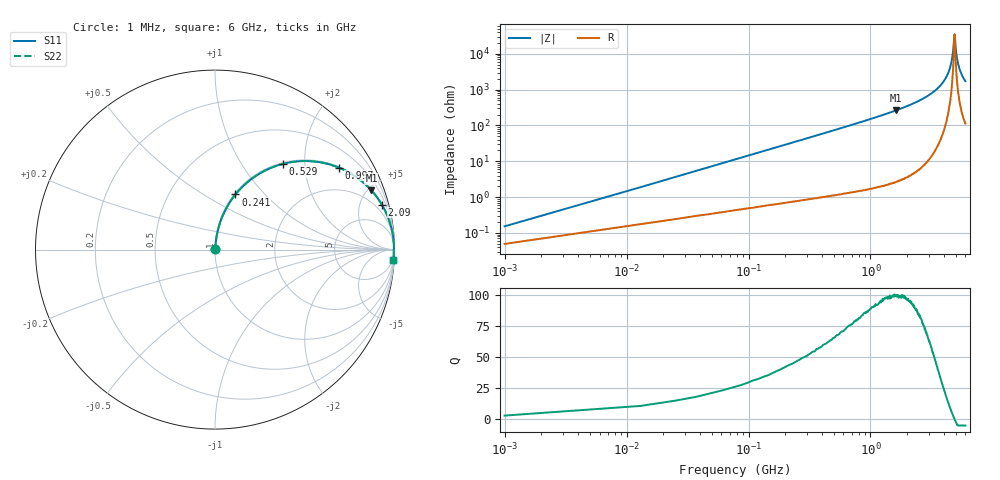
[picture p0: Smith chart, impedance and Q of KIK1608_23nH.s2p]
!version-2
!date-01.2022
!Series
# MHz S RI R 50
!Freq ReS11 ImS11 ReS21 ImS21 ReS12 ImS12 ReS22 ImS22
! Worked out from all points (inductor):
!   501 points, 1 MHz to 6 GHz, reference 50 ohm
!   read as one part in series: L = 23 nH near 25 MHz
!   highest Q = 99.8 at 1.62 GHz (marker M1), where L = 25.8 nH
!   self-resonance near 4.89 GHz
!   S11 on the Smith chart (normalised r, x): 1 MHz: 1.00, +0.00; 241 MHz: 1.02, +0.70; 529 MHz: 1.02, +1.55; 997 MHz: 1.03, +3.01; 2.09 GHz: 1.08, +7.38; 6 GHz: 3, -34
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1  0.00049 0.00144  0.9995 -0.00144  0.9995 -0.00144  0.00049 0.00144
37  0.00578 0.053  0.9942 -0.053  0.9942 -0.053  0.00578 0.053
61  0.0114 0.0868  0.9886 -0.0868  0.9886 -0.0868  0.0114 0.0868
133  0.0407 0.1835  0.9593 -0.1835  0.9593 -0.1835  0.0407 0.1835
241  0.1139 0.307  0.8861 -0.307  0.8861 -0.307  0.1139 0.307
529  0.3762 0.4771  0.6238 -0.4771  0.6238 -0.4771  0.3762 0.4771
997  0.6912 0.4564  0.3088 -0.4564  0.3088 -0.4564  0.6912 0.4564
1010  0.6967 0.4541  0.3033 -0.4541  0.3033 -0.4541  0.6967 0.4541
1620  0.8713 0.3299  0.1287 -0.3299  0.1287 -0.3299  0.8713 0.3299
2020  0.9227 0.262  0.0773 -0.262  0.0773 -0.262  0.9227 0.262
2090  0.9294 0.251  0.0706 -0.251  0.0706 -0.251  0.9294 0.251
3010  0.978 0.1391  0.022 -0.1391  0.022 -0.1391  0.978 0.1391
4010  0.9944 0.0563  0.00558 -0.0563  0.00558 -0.0563  0.9944 0.0563
4350  0.9963 0.0335  0.00367 -0.0335  0.00367 -0.0335  0.9963 0.0335
4590  0.997 0.0184  0.00302 -0.0184  0.00302 -0.0184  0.997 0.0184
4770  0.9972 0.00751  0.00285 -0.00751  0.00285 -0.00751  0.9972 0.00751
4890  0.9971 0.000523  0.00287 -0.000523  0.00287 -0.000523  0.9971 0.000523
4910  0.9971 -0.000855  0.00289 0.000855  0.00289 0.000855  0.9971 -0.000855
5010  0.997 -0.0063  0.003 0.0063  0.003 0.0063  0.997 -0.0063
5120  0.9968 -0.013  0.00321 0.013  0.00321 0.013  0.9968 -0.013
5360  0.9961 -0.0258  0.0039 0.0258  0.0039 0.0258  0.9961 -0.0258
6000  0.9929 -0.0574  0.00711 0.0574  0.00711 0.0574  0.9929 -0.0574
